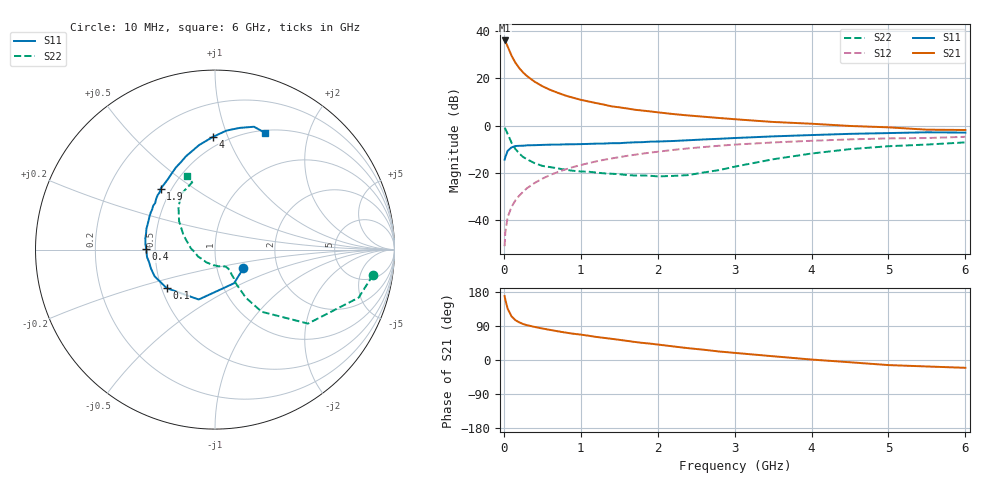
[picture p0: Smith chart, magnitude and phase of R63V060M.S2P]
! SIEMENS Small Signal Semiconductors
! BFR193
! Si NPN RF Bipolar Junction Transistor in SOT23
! VCE = 3 V  IC = 60 mA
! Common Emitter S-Parameters:  May  1996
# GHz  S  MA  R  50
!  f  S11  S21  S12  S22
! GHz  MAG  ANG  MAG  ANG  MAG  ANG  MAG  ANG
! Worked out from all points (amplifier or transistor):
!   36 points, 10 MHz to 6 GHz, reference 50 ohm
!   highest |S21| = 36.0 dB at 10 MHz (marker M1)
!   |S21| within 3 dB of that: start of sweep to 55.39 MHz
!   unconditionally stable (mu >= 1): 341 MHz to 1.846 GHz
!   at 250 MHz: K = 0.98, MSG = 25.3 dB, |S12| = -28.0 dB
!   at 1.4 GHz: K = 1.03, MAG = 10.0 dB, |S12| = -14.0 dB
!   at 6 GHz: K = 0.96, MSG = 1.4 dB, |S12| = -4.8 dB
!   S11 on the Smith chart (normalised r, x): 10 MHz: 1.34, -0.29; 100 MHz: 0.53, -0.26; 400 MHz: 0.45, +0.00; 1.9 GHz: 0.44, +0.37; 4 GHz: 0.43, +0.89; 6 GHz: 0.53, +1.38
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0.01  0.1892 -33.2  63.02 168.8  0.0028 80.2  0.8917 -9.1
0.02  0.2155 -60.5  60.12 158.4  0.0056 79.7  0.8437 -18.5
0.05  0.2926 -108.1  46.79 135.1  0.0116 71.4  0.6621 -38.5
0.1  0.3444 -141.5  30.05 115.2  0.0189 71.3  0.4332 -53.1
0.15  0.3679 -156.1  21.34 105.1  0.026 71.5  0.319 -57.3
0.2  0.3721 -163.5  16.41 99.3  0.0328 73.3  0.2577 -57.9
0.25  0.3739 -169.3  13.27 95.0  0.0396 74.0  0.2156 -58.4
0.3  0.381 -173.7  11.15 91.9  0.0471 75.2  0.194 -56.8
0.4  0.3837 179.4  8.449 87.3  0.0609 75.6  0.1599 -56.0
0.5  0.3888 175.3  6.796 83.1  0.0749 75.2  0.1399 -54.5
0.6  0.3933 170.7  5.698 79.5  0.0894 74.0  0.132 -55.0
0.7  0.3942 167.1  4.931 75.8  0.1037 73.3  0.124 -55.7
0.9  0.4007 159.5  3.87 69.4  0.132 70.8  0.1101 -58.9
1.1  0.4082 153.6  3.23 64.1  0.16 68.0  0.1053 -64.2
1.4  0.4226 144.6  2.544 55.9  0.2006 63.8  0.0954 -76.3
1.9  0.4552 131.7  1.991 43.3  0.2664 56.1  0.0865 -105.0
2.2  0.4701 124.4  1.749 35.9  0.3043 51.4  0.0858 -125.2
3.5  0.5888 98.7  1.189 9.9  0.438 30.5  0.1931 155.4
4  0.6279 91.1  1.09 1.2  0.4751 23.3  0.2555 141.6
4.5  0.6662 84.5  0.978 -6.0  0.5087 16.3  0.3165 130.0
5.5  0.7182 72.4  0.816 -17.1  0.5435 2.5  0.3957 108.7
6  0.7078 66.8  0.804 -20.6  0.5768 -1.5  0.4392 110.7
